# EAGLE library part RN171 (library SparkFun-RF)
Roving Networks RN-171 802.11b/g WiFi Serial Module The RN-171 is a small form factor, ultra-low power embedded TCP/IP module. The RN-171 is a standalone, complete TCP/IP wireless networking module. Due to its small form factor and extremely low power consumption, it is perfect for mobile wireless applications such as asset monitoring, sensors, and portable battery operated devices. SparkFun Products WiFly RN-171 802.11b/g Serial Module (WRL-11049)
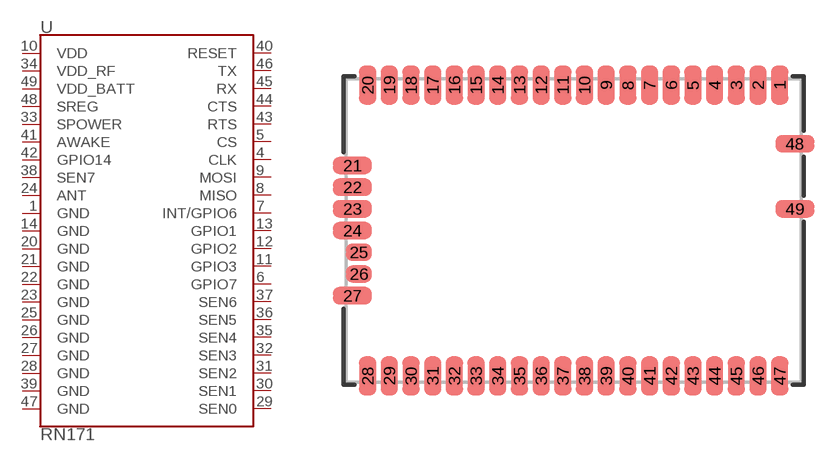
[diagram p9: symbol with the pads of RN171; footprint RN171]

Designator prefix U

## RN171 (PROD_ID: IC-11000; SF_ID: WRL-11049)  [RN171]
1  GND
4  CLK
5  CS
6  GPIO7
7  INT/GPIO6
8  MISO
9  MOSI
10  VDD
11  GPIO3
12  GPIO2
13  GPIO1
14  GND
20  GND
21  GND
22  GND
23  GND
24  ANT
25  GND
26  GND
27  GND
28  GND
29  SEN0
30  SEN1
31  SEN2
32  SEN3
33  SPOWER
34  VDD_RF
35  SEN4
36  SEN5
37  SEN6
38  SEN7
39  GND
40  RESET
41  AWAKE
42  GPIO14
43  RTS
44  CTS
45  RX
46  TX
47  GND
48  SREG
49  VDD_BATT

## Footprint RN171 (pad centres in mm)
Roving Networks RN-171 Wi-Fi Module 26.67 x 17.78 x 3.18 mm module Datasheet
smd 1.016 x 2.286: 1 12.065,8.509; 2 10.795,8.509; 3 9.525,8.509; 4 8.255,8.509; 5 6.985,8.509; 6 5.715,8.509; 7 4.445,8.509; 8 3.175,8.509; 9 1.905,8.509; 10 0.635,8.509; 11 -0.635,8.509; 12 -1.905,8.509; 13 -3.175,8.509; 14 -4.445,8.509; 15 -5.715,8.509; 16 -6.985,8.509; 17 -8.255,8.509; 18 -9.525,8.509; 19 -10.795,8.509; 20 -12.065,8.509; 28 -12.065,-8.509; 29 -10.795,-8.509; 30 -9.525,-8.509; 31 -8.255,-8.509; 32 -6.985,-8.509; 33 -5.715,-8.509; 34 -4.445,-8.509; 35 -3.175,-8.509; 36 -1.905,-8.509; 37 -0.635,-8.509; 38 0.635,-8.509; 39 1.905,-8.509; 40 3.175,-8.509; 41 4.445,-8.509; 42 5.715,-8.509; 43 6.985,-8.509; 44 8.255,-8.509; 45 9.525,-8.509; 46 10.795,-8.509; 47 12.065,-8.509
smd 2.286 x 1.016: 21 -12.954,3.81; 22 -12.954,2.54; 23 -12.954,1.27; 24 -12.954,0; 27 -12.954,-3.81; 48 12.954,5.08; 49 12.954,1.27
smd 1.524 x 1.016: 25 -12.573,-1.27; 26 -12.573,-2.54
